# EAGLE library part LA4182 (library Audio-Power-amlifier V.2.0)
Built-in 2 channels enabling use in stereo and bridge amplifier applications. High output: 2.3 W/channel, VCC=9V,RL=4Ω, and 4.7 W/bridge, RL=8Ω. Minimum number of external parts required : 9 pcs. min. (Stereo/bridge). Small pop noise at the time of power supply ON/OFF due to built-in muting circuit. Good ripple rejection ratio due to built-in ripple filter. Soft tone at the time of output saturation. Good channel separation. Voltage gain fixed at 45 dB (Bridge: 51 dB). Variable voltage gain available with external resistor added. Easy to design radiator fin.
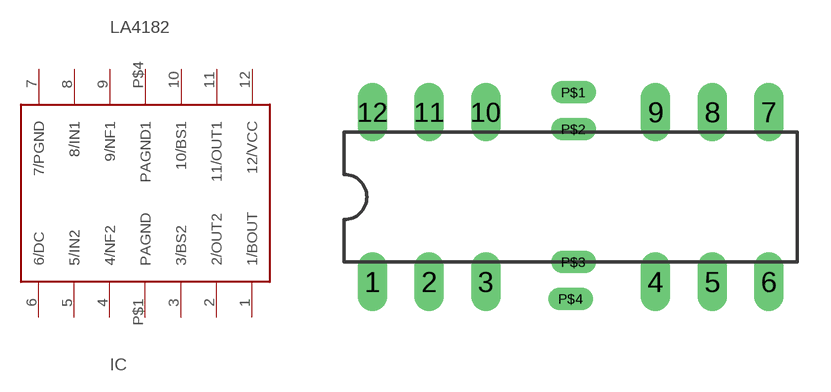
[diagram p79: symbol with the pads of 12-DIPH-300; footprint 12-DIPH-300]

Designator prefix IC

## LA4182  [12-DIPH-300]
1  1/BOUT
2  2/OUT2  out
3  3/BS2
4  4/NF2
5  5/IN2  in
6  6/DC
7  7/PGND  pwr
8  8/IN1  in
9  9/NF1
10  10/BS1
11  11/OUT1  out
12  12/VCC  pwr
P$1  PAGND  pwr
P$4  PAGND1  pwr

## Footprint 12-DIPH-300 (pad centres in mm)
Dual In Line Package
drill 0.813 long: 1 -8.89,-3.81; 2 -6.35,-3.81; 3 -3.81,-3.81; 4 3.81,-3.81; 5 6.35,-3.81; 6 8.89,-3.81; 7 8.89,3.81; 8 6.35,3.81; 9 3.81,3.81; 10 -3.81,3.81; 11 -6.35,3.81; 12 -8.89,3.81
drill 0.003 pad 1.016 long: P$1 0.127,4.699; P$2 0.127,3.048; P$3 0.127,-2.921; P$4 0,-4.572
